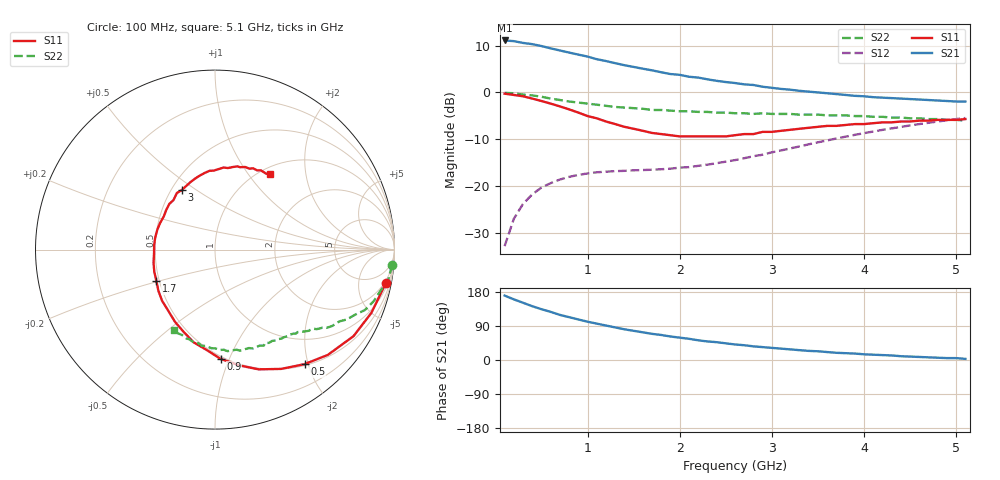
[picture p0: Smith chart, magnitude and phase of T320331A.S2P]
!AT-32033
!S and NOISE PARAMETERS at Vce=1V  Ic=1mA.  LAST UPDATED 01-05-95
# ghz s ma r 50
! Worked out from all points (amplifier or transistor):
!   51 points, 100 MHz to 5.1 GHz, reference 50 ohm
!   highest |S21| = 11.1 dB at 100 MHz (marker M1)
!   |S21| within 3 dB of that: start of sweep to 896.5 MHz
!   unconditionally stable (mu >= 1): 1.854 GHz to 3.114 GHz
!   at 900 MHz: K = 0.51, MSG = 12.8 dB, |S12| = -17.6 dB
!   at 2.6 GHz: K = 1.09, MAG = 6.4 dB, |S12| = -14.4 dB
!   at 5.1 GHz: K = 0.90, MSG = 1.8 dB, |S12| = -5.4 dB
!   lowest NFmin = 0.42 dB at 500 MHz
!   S11 on the Smith chart (normalised r, x): 100 MHz: 2, -10; 500 MHz: 0.52, -1.94; 900 MHz: 0.48, -0.93; 1.7 GHz: 0.48, -0.19; 3 GHz: 0.57, +0.44; 5.1 GHz: 1.11, +1.28
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0.1  0.97 -11.0  3.58 170.0  0.023 83.0  0.99 -5.0
0.2  0.94 -22.0  3.52 160.0  0.045 76.0  0.98 -10.0
0.3  0.91 -32.0  3.37 151.0  0.065 70.0  0.95 -14.0
0.4  0.86 -43.0  3.27 142.0  0.082 65.0  0.93 -18.0
0.5  0.81 -52.0  3.12 134.0  0.097 60.0  0.9 -22.0
0.7  0.71 -70.0  2.8 119.0  0.118 51.0  0.83 -28.0
0.9  0.61 -87.0  2.53 107.0  0.132 46.0  0.78 -33.0
1  0.56 -95.0  2.41 101.0  0.137 44.0  0.76 -35.0
1.2  0.49 -111.0  2.16 91.0  0.143 41.0  0.72 -38.0
1.4  0.43 -127.0  1.95 81.0  0.146 39.0  0.69 -41.0
1.7  0.37 -152.0  1.72 69.0  0.15 40.0  0.65 -45.0
1.8  0.36 -160.0  1.64 66.0  0.152 41.0  0.65 -46.0
1.9  0.35 -168.0  1.57 62.0  0.154 42.0  0.64 -47.0
2  0.34 -177.0  1.54 59.0  0.158 44.0  0.63 -49.0
2.2  0.34 169.0  1.44 52.0  0.165 46.0  0.62 -52.0
2.6  0.35 141.0  1.26 41.0  0.19 52.0  0.6 -58.0
2.8  0.36 130.0  1.2 36.0  0.209 53.0  0.59 -62.0
3  0.38 119.0  1.12 32.0  0.23 55.0  0.59 -65.0
3.5  0.43 98.0  1 23.0  0.294 54.0  0.58 -76.0
3.7  0.44 91.0  0.96 19.0  0.323 53.0  0.57 -80.0
4.3  0.48 73.0  0.87 12.0  0.414 47.0  0.54 -95.0
5.1  0.52 54.0  0.8 3.0  0.534 35.0  0.5 -117.0
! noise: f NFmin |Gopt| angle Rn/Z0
0.5  0.42  0.87  25  0.48
0.9  0.71  0.73  55  0.34
1.8  1.37  0.42  143  0.11
2.4  1.8  0.5  -162  0.07
